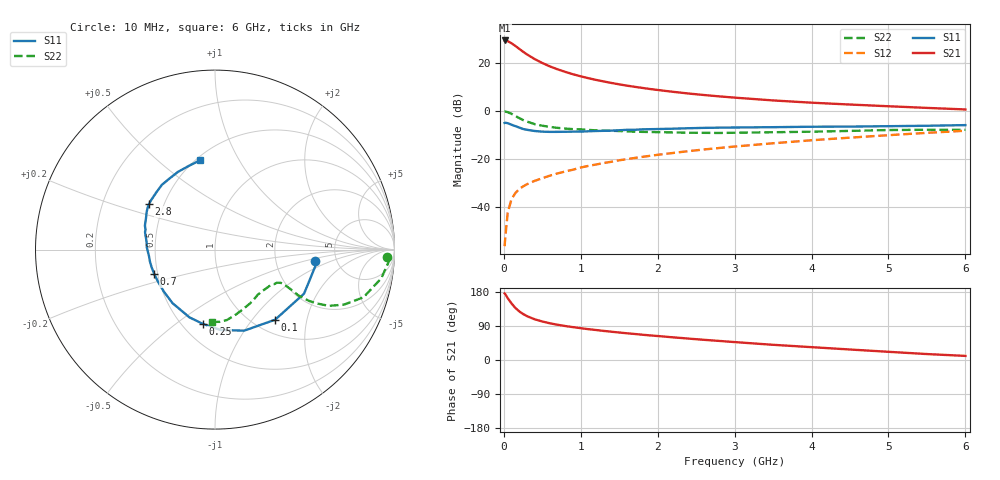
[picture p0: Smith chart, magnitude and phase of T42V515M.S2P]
! Infineon Technologies  Discrete & RF Semiconductors
! BFR182T
! Si NPN RF Bipolar Junction Transistor in SC75
! VCE = 2.5 V  IC = 15 mA
! Common Emitter S-Parameters:  October  1999
# GHz  S  MA  R  50
!  f  S11  S21  S12  S22
! GHz  MAG  ANG  MAG  ANG  MAG  ANG  MAG  ANG
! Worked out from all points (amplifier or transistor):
!   36 points, 10 MHz to 6 GHz, reference 50 ohm
!   highest |S21| = 29.4 dB at 10 MHz (marker M1)
!   |S21| within 3 dB of that: start of sweep to 179.3 MHz
!   unconditionally stable (mu >= 1): 746.5 MHz to 3.694 GHz
!   at 250 MHz: K = 0.58, MSG = 28.1 dB, |S12| = -31.5 dB
!   at 1.4 GHz: K = 1.11, MAG = 14.4 dB, |S12| = -21.2 dB
!   at 6 GHz: K = 0.84, MSG = 4.4 dB, |S12| = -8.3 dB
!   S11 on the Smith chart (normalised r, x): 10 MHz: 3.42, -0.63; 100 MHz: 1.24, -1.31; 250 MHz: 0.63, -0.63; 700 MHz: 0.48, -0.15; 2.8 GHz: 0.41, +0.26; 6 GHz: 0.52, +0.70
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0.01  0.5597 -6.5  29.52 175.6  0.0015 80.4  0.9608 -2.6
0.02  0.567 -9.2  29.41 173.4  0.0024 92.8  0.9703 -4.0
0.05  0.5536 -26.3  28.6 163.3  0.0075 82.8  0.9401 -9.8
0.1  0.5146 -49.4  25.79 149.2  0.0144 73.5  0.8692 -17.8
0.15  0.4801 -70.2  22.66 137.3  0.0193 65.4  0.7812 -23.1
0.2  0.4486 -86.2  19.75 128.4  0.0234 63.9  0.7075 -26.3
0.25  0.4189 -99.5  17.2 121.4  0.0265 61.5  0.6439 -27.8
0.3  0.4032 -110.8  15.13 115.8  0.0294 60.5  0.5984 -28.6
0.4  0.3807 -128.5  12.09 107.5  0.0346 61.4  0.5296 -28.8
0.5  0.3687 -140.5  9.992 101.6  0.0393 62.5  0.4904 -27.9
0.6  0.3644 -150.4  8.464 96.8  0.0445 63.6  0.4625 -27.4
0.7  0.365 -157.9  7.363 93.0  0.0497 65.2  0.4422 -27.0
0.9  0.3688 -169.9  5.81 86.7  0.0593 67.2  0.4154 -26.8
1.1  0.3752 -179.0  4.809 81.3  0.0712 68.1  0.4005 -27.5
1.3  0.3835 173.9  4.111 76.7  0.0817 69.0  0.3879 -28.8
1.6  0.4021 165.9  3.364 70.5  0.0983 69.3  0.3734 -31.3
2.2  0.4249 154.5  2.499 59.8  0.1324 69.1  0.3554 -38.5
2.8  0.4467 145.2  2.009 50.3  0.168 67.7  0.3463 -47.0
3.5  0.457 135.5  1.652 40.1  0.2109 65.1  0.3583 -57.4
4.5  0.4699 123.0  1.357 27.7  0.2764 60.0  0.382 -73.1
5.5  0.4892 107.1  1.155 15.7  0.3481 53.9  0.4034 -86.6
6  0.5047 99.4  1.072 10.8  0.3851 50.1  0.4025 -92.2
